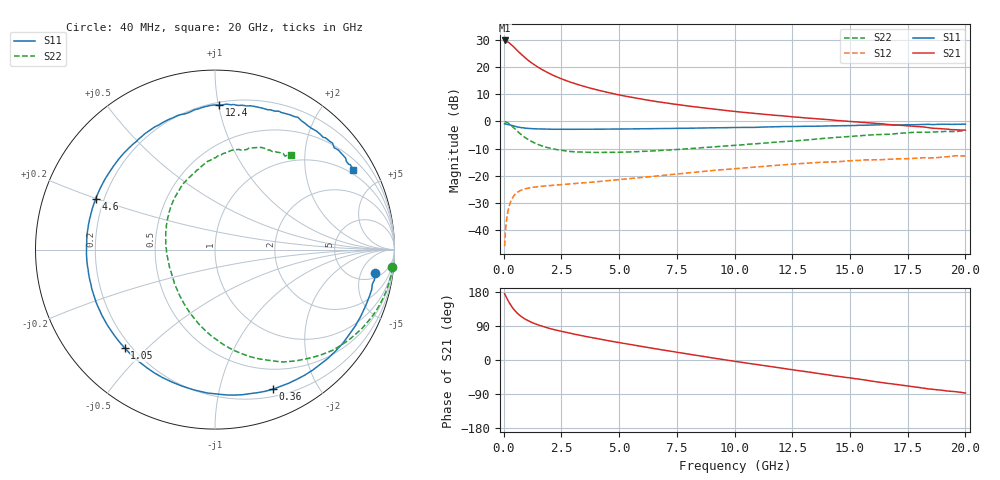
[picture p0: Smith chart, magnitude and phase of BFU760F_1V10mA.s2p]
! Filename:  P:\Prog\Test\Noise\ATS_data\Testdata_Net\Split files Spar\BFU760F_2W_C1_1V_5mA_60mA_Bias3_D.s2p
! Date/Time: Mon 06/Feb/2012 15:06:03
! BFU760_2W_C1_1V_5mA_60mA_Bias3_R.s2p
! MDIF S-parameter v. bias file
! BFU760_2W_C1_1V_5mA_60mA
! Date/time Fri Mar 18 10:56:44 2011
! VAR V_out= 1.0001
! VAR I_out= 10.0600
! VAR V_in= 0.7770
! VAR I_in= 0.0293
! Device data file deembeded for feedlines and parallel
! Original file: \Split files Spar\BFU760_2W_C1_1V_5mA_60mA_Bias3_R.s2p
! Feed-files: PR003V01_101208_Feed1.s2p, PR003V01_101208_Feed2.s2p
! Parallel-file: PR003V01_101208_Par.s2p
# MHz S MA R 50
!  Freq-MHz  S11-mag  S11-arg  S21-mag  S21-arg  S12-mag  S12-arg  S22-mag  S22-arg
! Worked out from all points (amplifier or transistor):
!   167 points, 40 MHz to 20 GHz, reference 50 ohm
!   highest |S21| = 29.8 dB at 40 MHz (marker M1)
!   |S21| within 3 dB of that: start of sweep to 509.9 MHz
!   unconditionally stable (mu >= 1): 5.19 GHz to 14.85 GHz
!   at 550 MHz: K = 0.13, MSG = 26.4 dB, |S12| = -26.4 dB
!   at 4.2 GHz: K = 0.89, MSG = 16.7 dB, |S12| = -22.1 dB
!   at 20 GHz: K = 0.88, MSG = 4.7 dB, |S12| = -12.7 dB
!   S11 on the Smith chart (normalised r, x): 40 MHz: 7, -9; 360 MHz: 0.27, -1.46; 1.05 GHz: 0.17, -0.43; 4.6 GHz: 0.17, +0.20; 12.4 GHz: 0.22, +1.00; 20 GHz: 0.82, +3.56
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40  0.9031 -8.3  30.83 175.1  0.005073 85.4  0.9934 -5.7
50  0.9038 -10.8  30.8 173.2  0.006162 87.9  0.9911 -7.2
120  0.8931 -24.6  29.97 164.8  0.01492 77.4  0.9716 -17.2
220  0.8737 -43.9  28.23 153.4  0.02591 67.6  0.9162 -30.6
280  0.8597 -54.5  26.92 147.3  0.03155 62.3  0.877 -37.9
360  0.8421 -67.5  25.08 140.1  0.03773 56.0  0.8156 -47.0
460  0.8181 -82.2  22.96 132.0  0.04387 49.5  0.7458 -56.7
550  0.8 -93.1  21.03 125.9  0.0478 44.8  0.6825 -64.5
650  0.7826 -103.5  19.04 120.1  0.05136 40.3  0.6262 -72.0
850  0.7597 -120.1  15.82 111.0  0.05612 34.0  0.5342 -84.6
1050  0.744 -132.5  13.42 104.0  0.05905 29.9  0.4665 -94.8
1400  0.7299 -148.0  10.49 94.7  0.06241 25.4  0.3903 -109.2
1850  0.7207 -161.5  8.123 85.6  0.06525 22.5  0.3342 -123.7
2500  0.7166 -175.0  6.072 75.6  0.06867 20.9  0.2947 -140.1
3400  0.7175 171.4  4.51 64.1  0.07382 19.9  0.2731 -156.8
4600  0.723 156.9  3.343 50.2  0.08193 19.4  0.2686 -174.9
6800  0.7372 135.2  2.258 27.4  0.1006 16.4  0.2921 159.6
10200  0.7746 106.1  1.496 -5.2  0.1373 4.8  0.3696 126.8
12400  0.8045 88.4  1.23 -24.8  0.1628 -5.9  0.4326 107.8
13400  0.8132 81.0  1.131 -33.5  0.174 -12.4  0.4667 99.8
16800  0.8641 54.6  0.8682 -62.8  0.2017 -32.7  0.585 72.4
20000  0.891 30.0  0.6909 -87.2  0.2323 -53.9  0.6732 51.1
